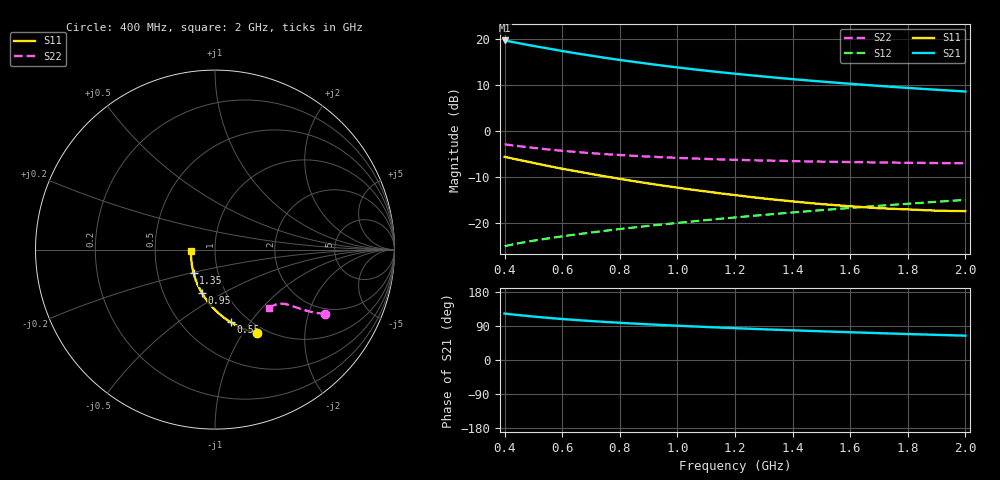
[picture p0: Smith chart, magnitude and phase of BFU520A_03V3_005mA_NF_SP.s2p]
! Filename:  P:\Prog\Test\Noise\ATS_data\Testdata_Net\06 Compressed Noise after Statistics\BFU520A_APG2013_30_A05_03p3V_005mA_NF_CM01_D.sf
! Date/Time: Wed 24/Apr/2013 20:06:16
! BFU520A_APG2013_30_A05_03p3V_1to20mA_NF_CM01_Bias4_R.sf
! Noise Parameter Data File
! BFU520A_APG2013_30_A05_03p3V_1to20mA_NF_CM01
! Date/time: Thu Apr 11 00:04:13 2013
! VAR V_out= 3.301000
! VAR I_out= 5.000000
! VAR V_in= 0.832700
! VAR I_in= 0.055610
! Device data file deembeded for feedlines and parallel
! Original file: \06 Compressed Noise after Statistics\BFU520A_APG2013_30_A05_03p3V_005mA_NF_CM01_R.sf
! Feed-files: PR017V01_150413_Feed1.s2p, PR017V01_150413_Feed2.s2p
! Parallel-file: PR017V01_150413_Par.s2p
# MHz S MA R 50
!  Freq-MHz  S11-mag  S11-arg  S21-mag  S21-arg  S12-mag  S12-arg  S22-mag  S22-arg
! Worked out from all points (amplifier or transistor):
!   37 points, 400 MHz to 2 GHz, reference 50 ohm
!   highest |S21| = 19.6 dB at 400 MHz (marker M1)
!   |S21| within 3 dB of that: start of sweep to 668.7 MHz
!   unconditionally stable (mu >= 1): 1.585 GHz to end of sweep
!   at 500 MHz: K = 0.63, MSG = 21.2 dB, |S12| = -23.9 dB
!   at 1.1 GHz: K = 0.93, MSG = 16.3 dB, |S12| = -19.5 dB
!   at 2 GHz: K = 1.01, MAG = 11.1 dB, |S12| = -15.1 dB
!   lowest NFmin = 0.64 dB at 420 MHz
!   S11 on the Smith chart (normalised r, x): 400 MHz: 0.91, -1.15; 550 MHz: 0.83, -0.81; 950 MHz: 0.77, -0.40; 1.35 GHz: 0.76, -0.20; 2 GHz: 0.76, -0.01
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400  0.5197 -63.4  9.601 122.6  0.05542 64.1  0.7106 -30.1
420  0.5044 -65.6  9.336 120.8  0.05721 63.7  0.6975 -30.7
440  0.4884 -67.7  9.086 119.2  0.05886 63.4  0.6852 -31.2
480  0.4606 -71.5  8.592 116.2  0.06204 62.9  0.6616 -32.1
500  0.4465 -73.4  8.368 114.7  0.0636 62.7  0.6514 -32.5
550  0.4142 -77.9  7.864 111.2  0.06724 62.4  0.6256 -33.3
600  0.3857 -82.0  7.372 108.2  0.0709 62.3  0.6048 -34.0
650  0.3617 -85.7  6.942 105.4  0.07449 62.2  0.5866 -34.6
700  0.3388 -89.5  6.56 102.8  0.07803 62.3  0.5703 -35.0
750  0.3181 -93.0  6.206 100.5  0.08156 62.4  0.556 -35.4
800  0.2999 -96.6  5.893 98.2  0.08511 62.6  0.5438 -35.8
850  0.2823 -100.0  5.606 96.1  0.08862 62.8  0.5326 -36.2
900  0.2669 -103.5  5.346 94.1  0.09218 62.9  0.5229 -36.6
950  0.2527 -106.6  5.104 92.2  0.09569 63.1  0.5141 -36.9
1050  0.2284 -113.0  4.683 88.8  0.1028 63.6  0.4991 -37.5
1100  0.2182 -116.4  4.499 87.1  0.1065 63.8  0.4933 -37.9
1200  0.1994 -122.8  4.172 84.0  0.1138 64.1  0.4826 -38.6
1350  0.1764 -132.6  3.761 79.7  0.1251 64.4  0.4706 -39.9
1500  0.1592 -142.9  3.429 75.8  0.1365 64.6  0.4605 -41.3
1650  0.147 -153.0  3.157 72.0  0.1484 64.7  0.4539 -42.9
1750  0.1413 -160.1  2.997 69.7  0.1563 64.7  0.4495 -44.0
2000  0.1335 -176.6  2.672 64.2  0.1768 64.4  0.4423 -47.1
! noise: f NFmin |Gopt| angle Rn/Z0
400  0.6997  0.1928  14.34  0.1279
460  0.6826  0.1726  20.23  0.1204
600  0.7721  0.188  21.75  0.1346
800  0.7388  0.1445  44.32  0.1095
1000  0.7591  0.1466  57.86  0.1055
1200  0.801  0.1314  67.75  0.1065
1400  0.8363  0.1308  87.87  0.0987
1600  0.8629  0.1341  118.4  0.0778
1800  0.807  0.1479  143.9  0.074
2000  0.866  0.1236  139.9  0.0794
